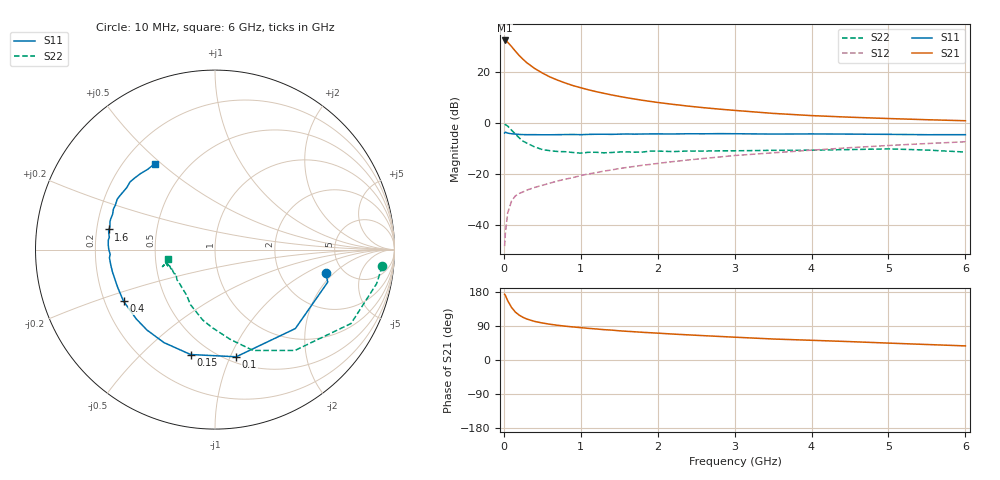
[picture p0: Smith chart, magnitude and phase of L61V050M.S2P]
!  INFINEON TECHNOLOGIES Small Signal Semiconductors
! BFR380L3 , Si-NPN RF-Transistor in TSLP-3-1
!  Vce=1 V,  Ic=50 mA
! Common Emitter S-Parameters:  07. March 2005
#  GHz  S  MA  R  50
! f  S11  S21  S12  S22
! GHz  Mag  Ang  Mag  Ang  Mag  Ang  Mag  Ang
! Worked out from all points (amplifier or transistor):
!   36 points, 10 MHz to 6 GHz, reference 50 ohm
!   highest |S21| = 32.3 dB at 10 MHz (marker M1)
!   |S21| within 3 dB of that: start of sweep to 117.1 MHz
!   unconditionally stable (mu >= 1): 1.285 GHz to 5.672 GHz
!   at 250 MHz: K = 0.49, MSG = 26.0 dB, |S12| = -27.1 dB
!   at 1.4 GHz: K = 1.02, MAG = 13.9 dB, |S12| = -18.5 dB
!   at 6 GHz: K = 1.00, MSG = 4.1 dB, |S12| = -7.4 dB
!   S11 on the Smith chart (normalised r, x): 10 MHz: 3.68, -1.59; 100 MHz: 0.56, -1.05; 150 MHz: 0.39, -0.72; 400 MHz: 0.28, -0.24; 1.6 GHz: 0.25, +0.09; 6 GHz: 0.33, +0.47
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0.01  0.6308 -11.9  41.21 173.4  0.0038 72.5  0.9358 -5.7
0.02  0.6538 -16.1  40.96 170.5  0.0068 78.3  0.9203 -11.9
0.05  0.6277 -44.5  38.01 156.5  0.017 70.2  0.8627 -28.5
0.1  0.6087 -78.8  31.36 138.7  0.0292 59.9  0.717 -51.6
0.15  0.6002 -103.1  25.38 126.4  0.0368 52.2  0.6009 -69.3
0.2  0.591 -118.7  20.85 118.3  0.0411 50.2  0.5063 -80.5
0.25  0.587 -130.2  17.58 112.5  0.044 48.1  0.436 -91.8
0.3  0.5845 -138.5  15.01 108.1  0.0479 48.5  0.3992 -99.7
0.4  0.5851 -150.6  11.65 101.8  0.0539 50.0  0.3359 -114.0
0.5  0.5816 -158.5  9.477 97.7  0.0594 51.7  0.2986 -122.1
0.6  0.5819 -163.9  7.922 94.3  0.0655 53.9  0.2836 -129.3
0.7  0.5849 -167.8  6.856 91.6  0.0723 56.3  0.2735 -136.0
0.9  0.5899 -175.6  5.361 87.2  0.0843 59.1  0.2612 -145.7
1.1  0.5919 179.8  4.437 83.5  0.0993 61.0  0.2639 -149.5
1.3  0.5967 174.9  3.789 80.1  0.1127 62.0  0.2576 -155.9
1.6  0.6032 169.3  3.097 75.7  0.133 63.2  0.2689 -160.0
2.2  0.6036 160.9  2.299 68.4  0.1733 63.8  0.2723 -161.2
2.8  0.6128 152.8  1.854 62.2  0.213 63.6  0.282 -164.9
3.5  0.6008 144.9  1.529 55.4  0.2575 61.3  0.2883 -163.7
4.5  0.5998 138.5  1.287 48.5  0.325 59.1  0.2983 -162.8
5.5  0.5838 130.2  1.149 40.9  0.3914 54.7  0.2918 -163.7
6  0.5844 125.2  1.097 37.2  0.4243 52.3  0.2667 -168.2
